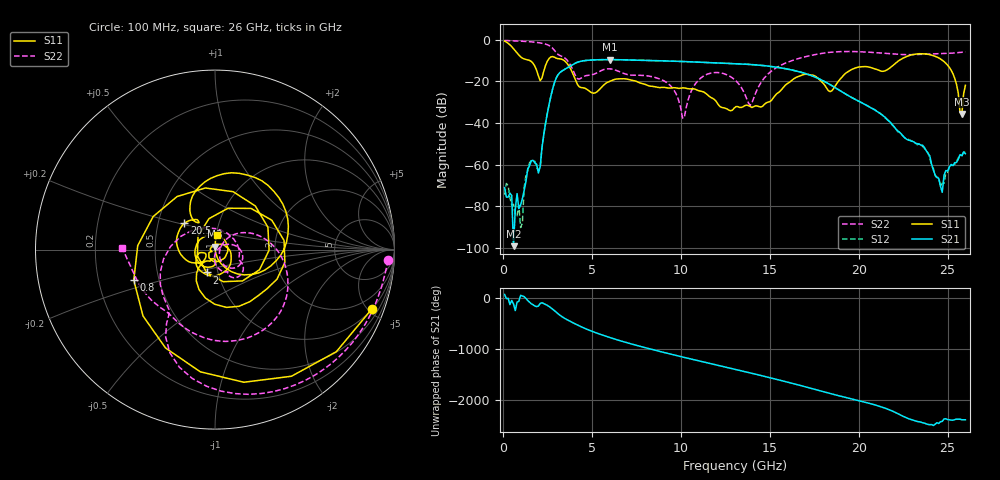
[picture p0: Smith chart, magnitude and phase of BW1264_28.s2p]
!Keysight Technologies,N5245B,MY57181159,A.13.60.06
!Date: Friday, December 18, 2020 23:53:24
!Correction: S11(Full 2 Port(1,2))
!S21(Full 2 Port(1,2))
!S12(Full 2 Port(1,2))
!S22(Full 2 Port(1,2))
!S2P File: Measurements: S11, S21, S12, S22:
# Hz S  dB  R 50
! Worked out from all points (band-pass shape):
!   260 points, 100 MHz to 26 GHz, reference 50 ohm
!   highest |S21| = -9.50 dB at 6 GHz (marker M1); lowest = -99.3 dB at 600 MHz (marker M2)
!   |S21| within 3 dB of the highest: 3.807 GHz to 14.78 GHz (10.97 GHz wide, 118 % of centre)
!   lowest |S11| = -35.7 dB at 25.8 GHz (marker M3), VSWR 1.03, Z = 50 + j1.64 ohm
!   |S11| at or under -10 dB: 1.52 GHz to 2.523 GHz (1.003 GHz wide, 49.6 % of centre); 3.45 GHz to 22.26 GHz (18.81 GHz wide, 146 % of centre); 24.73 GHz to end of sweep
!   |S22| runs from -37.6 to -0.3 dB; largest |S21 - S12| = 0.00069
!   S11 on the Smith chart (normalised r, x): 100 MHz: 1.01, -5.24; 800 MHz: 0.36, -0.16; 2 GHz: 0.88, -0.23; 20.5 GHz: 0.68, +0.21; 26 GHz: 1.01, +0.16
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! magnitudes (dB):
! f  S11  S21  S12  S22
! 100 MHz  -0.6  -71.1  -74.5  -0.3
! 600 MHz  -4.2  -99.3  -79.1  -0.5
! 800 MHz  -6.3  -74.0  -84.7  -0.6
! 1 GHz  -8.2  -79.5  -90.3  -0.6
! 1.5 GHz  -9.9  -60.6  -59.1  -0.9
! 2 GHz  -17.4  -64.0  -62.9  -1.4
! 3 GHz  -8.8  -18.4  -18.4  -6.1
! 4.5 GHz  -23.1  -10.1  -10.1  -17.9
! 6 GHz  -20.0  -9.5  -9.5  -14.0
! 8.8 GHz  -23.0  -10.1  -10.1  -18.8
! 10.1 GHz  -23.1  -10.4  -10.4  -37.6
! 11.2 GHz  -24.8  -10.8  -10.8  -17.9
! 13.1 GHz  -32.1  -11.5  -11.5  -19.7
! 13.9 GHz  -32.0  -11.9  -11.9  -31.5
! 17.4 GHz  -17.0  -17.4  -17.4  -7.4
! 18.4 GHz  -24.9  -21.6  -21.6  -6.0
! 20.5 GHz  -13.0  -31.8  -31.8  -5.9
! 21.7 GHz  -13.9  -39.1  -39.0  -6.6
! 23.7 GHz  -6.8  -51.8  -52.2  -6.9
! 24.7 GHz  -9.8  -73.3  -69.0  -6.6
! 25.8 GHz  -35.7  -55.7  -55.8  -6.0
! 26 GHz  -21.9  -54.8  -53.8  -5.7
